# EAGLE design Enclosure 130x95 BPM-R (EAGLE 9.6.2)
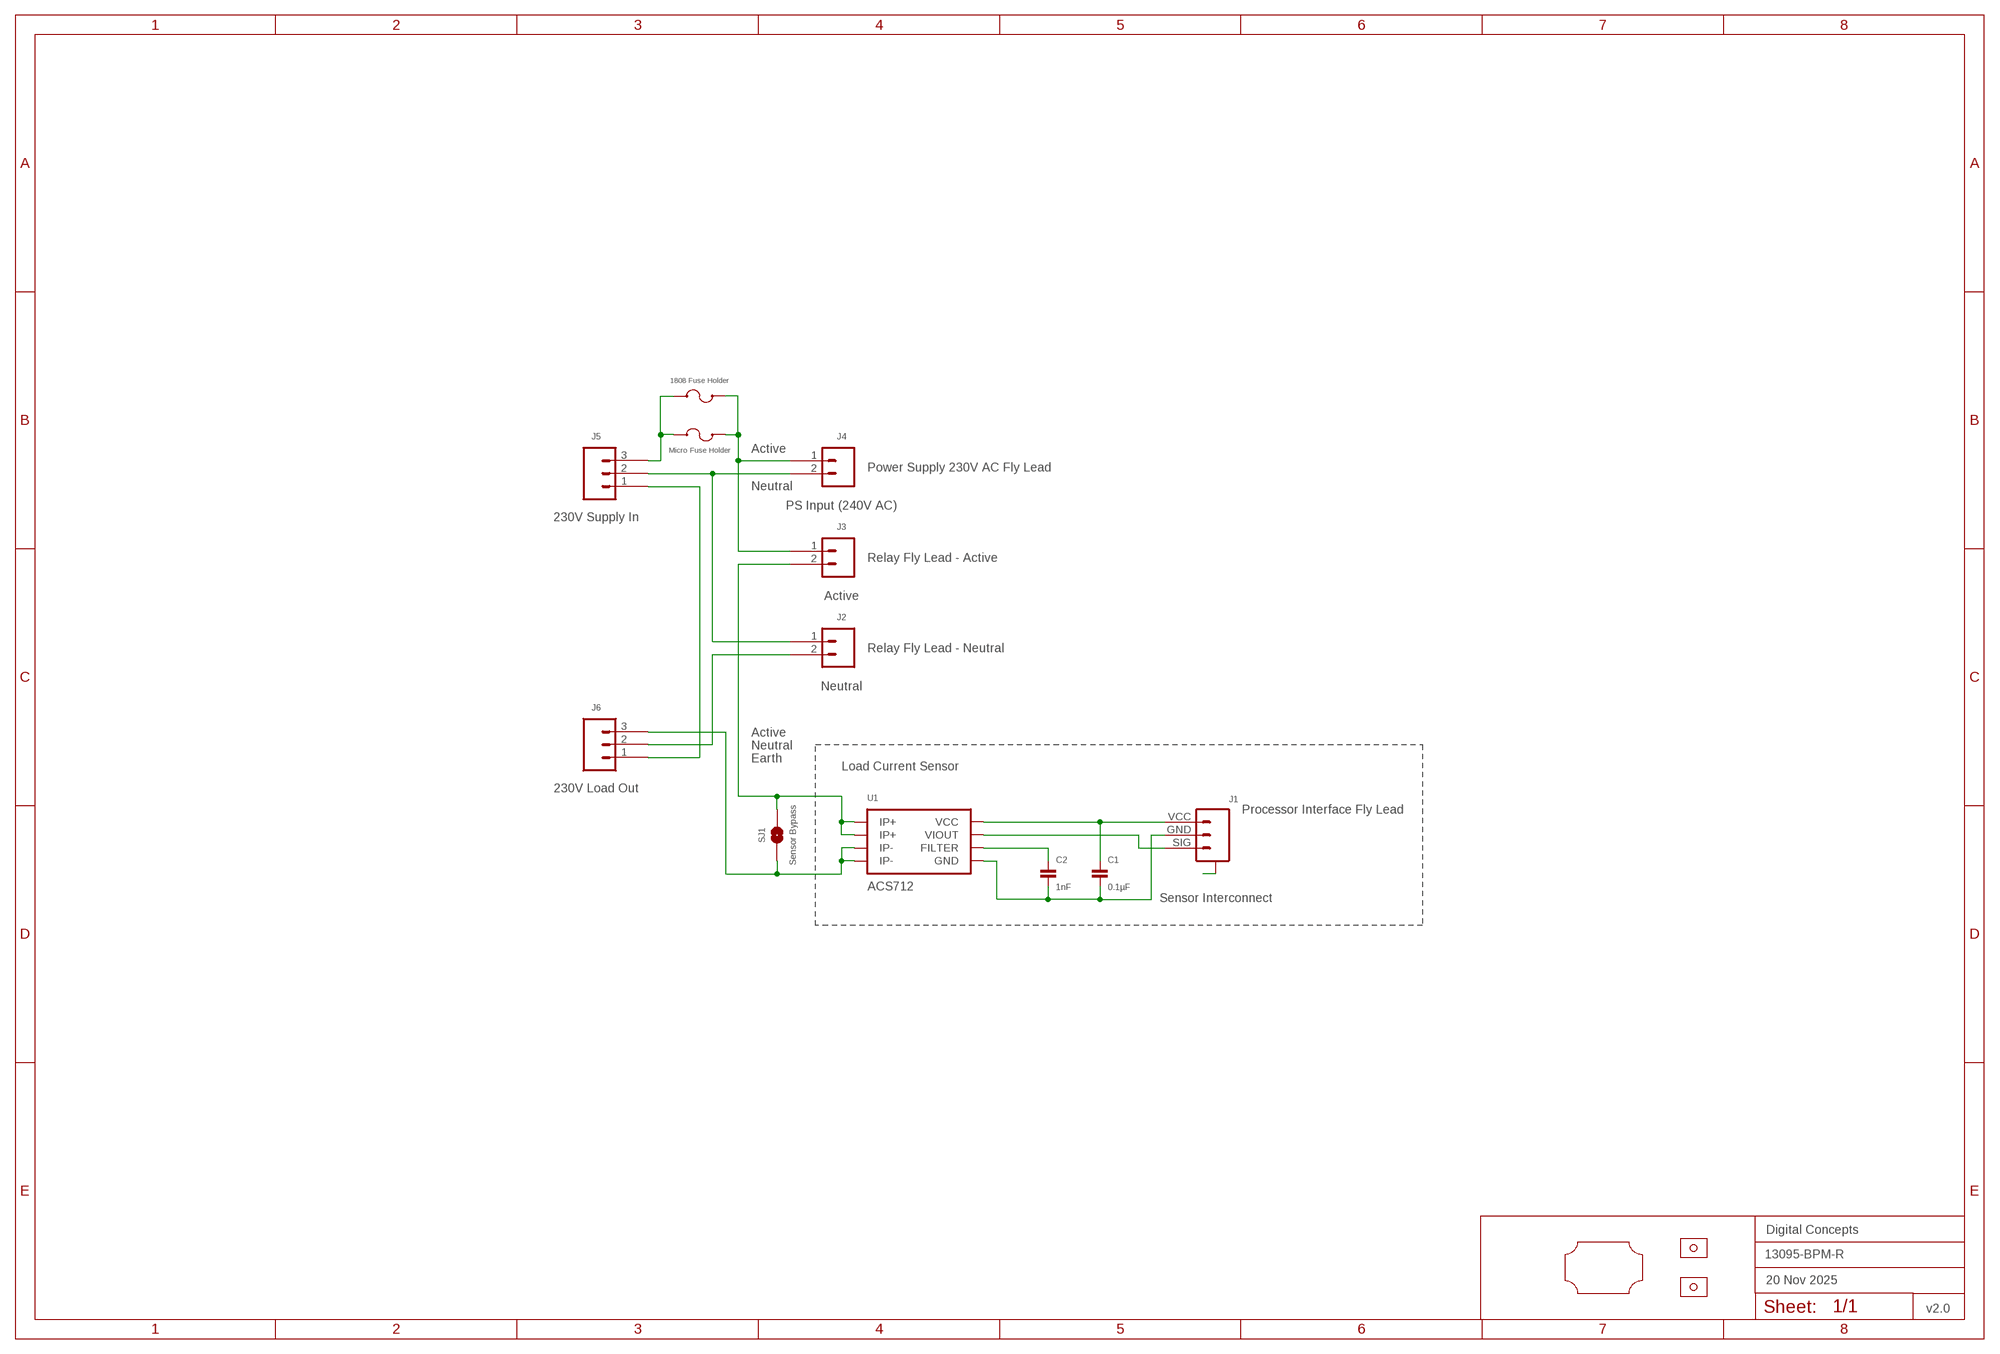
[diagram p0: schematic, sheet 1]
FRAME2 (A3L-LOC): DATE: 20 Nov 2025; OWNER: Digital Concepts; TITLE: 13095-BPM-R; VERSION: v2.0

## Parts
C1  0.1µF  CAPACITOR-0805  [C0805]
C2  1nF  CAPACITOR-0805  [C0805]
F2  1808 Fuse Holder  FUSE-HOLDER-1808  [FUSE-HOLDER-1808]
J1  Sensor Interconnect  JST-SH1.0-3-SMD-HORIZONTAL-SIG  [JST-SH1.0-3-HORIZONTAL-SIG]
J2  Neutral  TERMINAL_SCREW_2P_VERTICAL  [TERMINAL-SCREW-2P]
J3  Active  TERMINAL_SCREW_2P_VERTICAL  [TERMINAL-SCREW-2P]
J4  PS Input (240V AC)  JST-XH2.54-2-HORIZONTAL  [JST-XH2.4-2-HORIZONTAL]
J5  230V Supply In  TERMINAL_SCREW_3P_VERTICAL  [TERMINAL-SCREW-3P]
J6  230V Load Out  TERMINAL_SCREW_3P_VERTICAL  [TERMINAL-SCREW-3P]
SJ1  Sensor Bypass  SJ  [SJ]
U1  ACS712  [SOP-8]
U$1  PCB-OUTLINE-130X95-MAX-RC-H3  [PROTO-130X95-OUTLINE-MAX-RC-H3]
U$2  Micro Fuse Holder  FUSE-HOLDER  [FUSE-HOLDER-MICRO]
U$4  STRAIN-RELIEF-SADDLE  [STRAIN-RELIEF-SADDLE]
U$5  STRAIN-RELIEF-SADDLE  [STRAIN-RELIEF-SADDLE]

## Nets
A: J1.A@1(A) J1.A@3(A)
ACTIVE_IN: F2.P$2 J3.1 J4.1 U$2.P$3 U$2.P$4
ACTIVE_OUT: J3.2 SJ1.2 U1.1(IP+) U1.2(IP+)
EARTH: J5.1 J6.1
N$2: C1.1 J1.VCC U1.8(VCC)
N$3: J1.SIG U1.7(VIOUT)
N$7: F2.P$1 J5.3 U$2.P$1 U$2.P$2
N$19: J6.3 SJ1.1 U1.3(IP-) U1.4(IP-)
N$20: C1.2 C2.2 J1.GND U1.5(GND)
N$24: C2.1 U1.6(FILTER)
NEUTRAL_IN: J2.1 J4.2 J5.2
NEUTRAL_OUT: J2.2 J6.2

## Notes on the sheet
- Active
- Power Supply 230V AC Fly Lead
- Neutral
- Relay Fly Lead - Active
- Relay Fly Lead - Neutral
- Active
- Neutral
- Earth
- Load Current Sensor
- Processor Interface Fly Lead

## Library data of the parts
C1 C2 = digitalconcepts:CAPACITOR-0805: 0805 Capacitor
F2 = digitalconcepts:FUSE-HOLDER-1808: 1808 Fuse Holder
J1 = digitalconcepts:JST-SH1.0-3-SMD-HORIZONTAL-SIG: JST SH1.0 3P SMD Horizontal Connector with Signal
J2 J3 = digitalconcepts:TERMINAL_SCREW_2P_VERTICAL: PCB Mount Screw-Type Terminal 2P
J4 = digitalconcepts:JST-XH2.54-2-HORIZONTAL: XH2.54 2P Horizontal Connector
J5 J6 = digitalconcepts:TERMINAL_SCREW_3P_VERTICAL: PCB Mount Screw-Type Terminal 3P
SJ1 = digitalconcepts:SJ: Solder Jumper
U1 = digitalconcepts:ACS712: ACS712 Hall-Effect-Based Linear Current Sensor IC
U$1 = digitalconcepts:PCB-OUTLINE-130X95-MAX-RC-H3: PCB Eagle Max-Right-Cropped outline for 130 x 95 enclosure (Horizontal format)
U$2 = digitalconcepts:FUSE-HOLDER: Fuse Holder
U$4 U$5 = digitalconcepts:STRAIN-RELIEF-SADDLE: Strain Relief Saddle (7mm x 13mm)

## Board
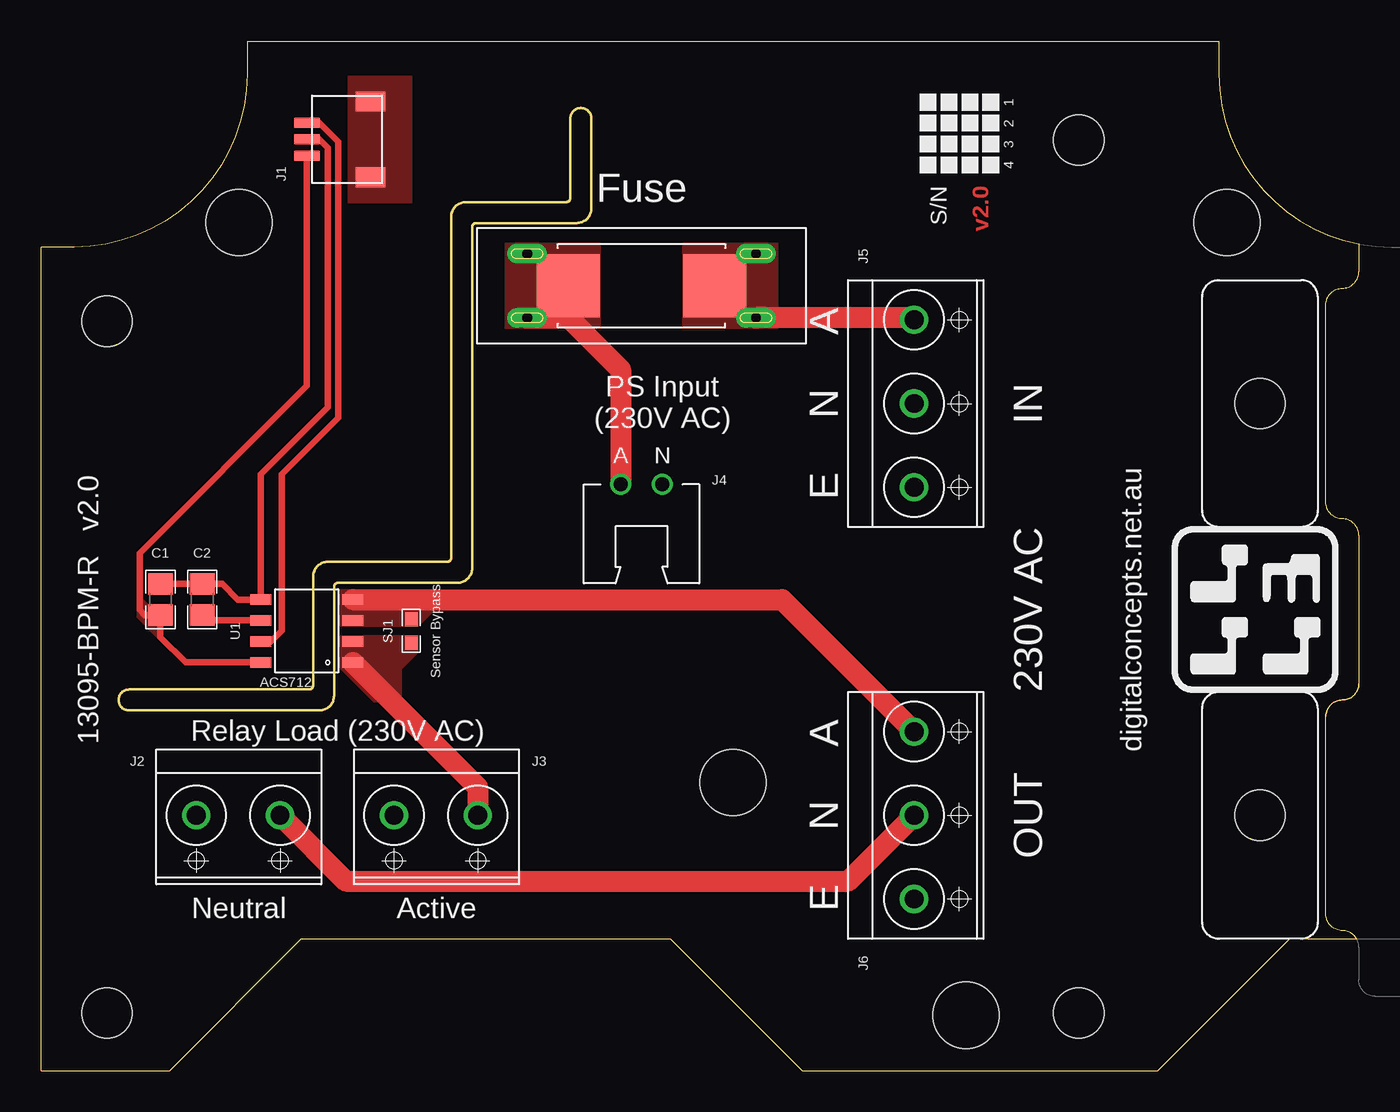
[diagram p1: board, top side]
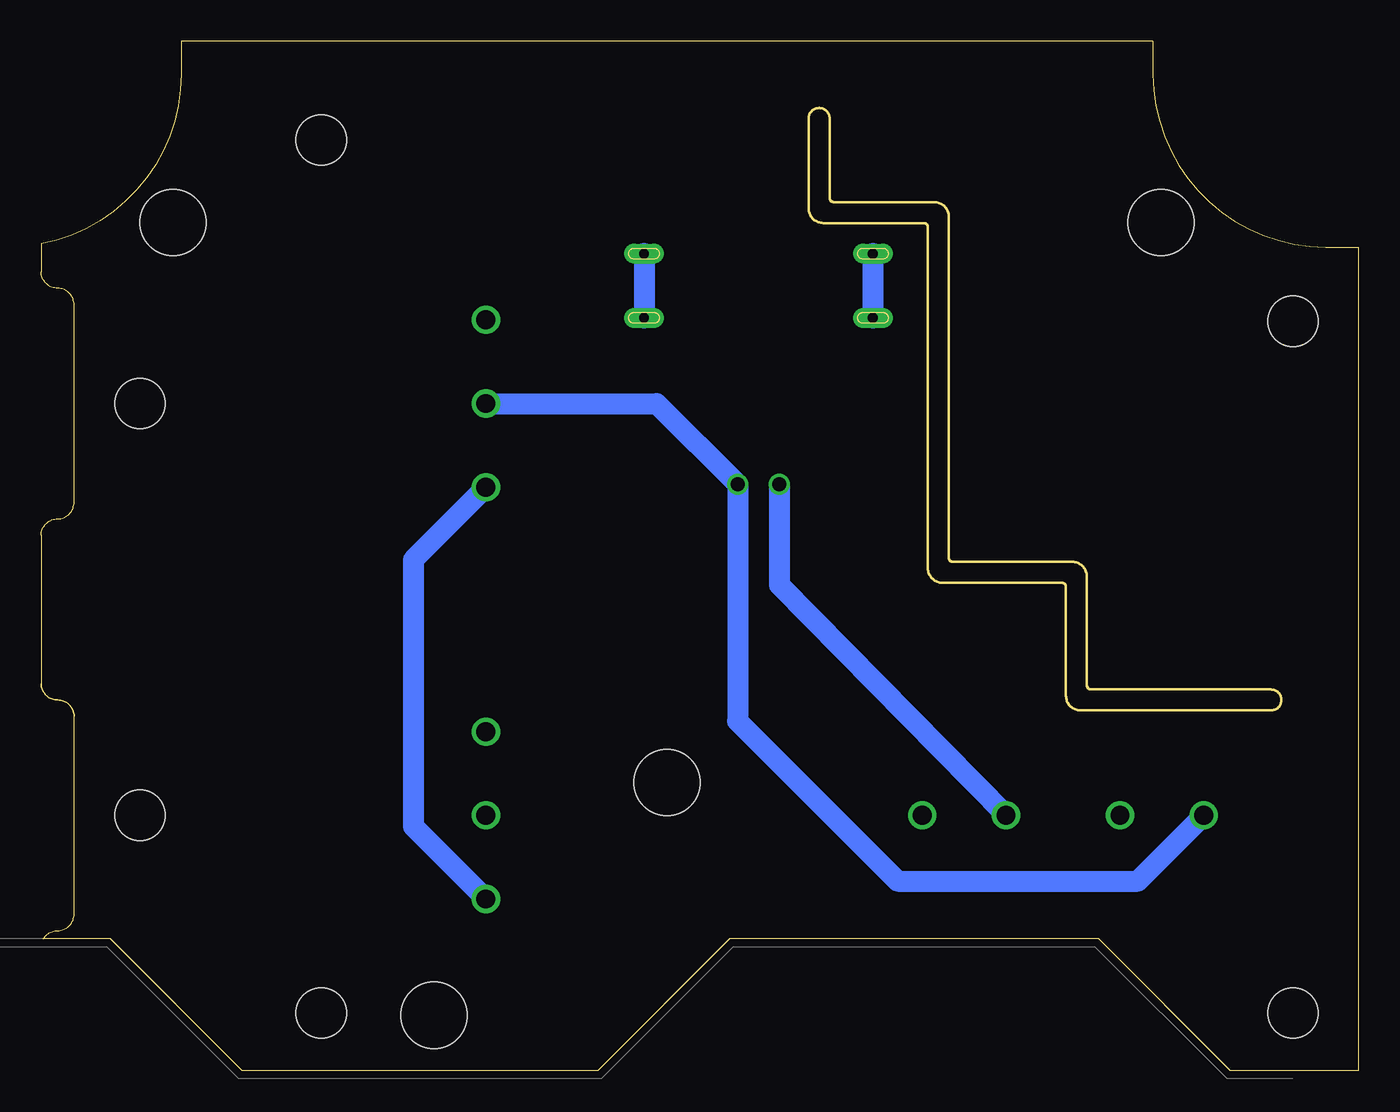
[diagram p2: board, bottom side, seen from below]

Size 80 x 62.5 mm. Coordinates in mm from the lower left corner, seen from the top.
Copper layers (1*16): Top 0.035mm / dielectric 1.5mm / Bottom 0.035mm
Design rules "default *": minimum track width 6mil, minimum drill 0.35mm, track to track 6mil, track to pad 6mil, pad to pad 6mil, via to via 6mil, smd to smd 6mil, copper to edge 6mil, drill to drill 6mil, minimum pad ring 1mil, minimum via ring 8mil, stop-mask expansion 4mil, vias tented up to drill 0mil, thermal gap 10mil
Milling: 24 lines

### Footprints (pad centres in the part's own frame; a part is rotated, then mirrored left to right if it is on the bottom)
C0805 = smd 1.3 x 1.5: 1 -0.95,0; 2 0.95,0
FUSE-HOLDER-1808 = smd 3.81 x 3.81: P$1 -4.445,0; P$2 4.445,0
JST-SH1.0-3-HORIZONTAL-SIG = smd 1.2 x 1.8: A@1 -2.3,-1.335; A@3 2.3,-1.335 | smd 0.6 x 1.55: GND 0,2.54; SIG 1,2.54; VCC -1,2.54
TERMINAL-SCREW-2P = drill 1.143: 1 -2.58,0; 2 2.5,0
JST-XH2.4-2-HORIZONTAL = drill 0.85: 1 1.27,0; 2 -1.27,0
TERMINAL-SCREW-3P = drill 1.143: 1 -5.08,0; 2 0,0; 3 5.08,0
SJ = smd 0.864 x 0.762: 1 -0.711,0; 2 0.711,0
SOP-8 = smd 0.635 x 1.27: 1 -1.905,-2.794; 2 -0.635,-2.794; 3 0.635,-2.794; 4 1.905,-2.794; 5 1.905,2.794; 6 0.635,2.794; 7 -0.635,2.794; 8 -1.905,2.794
PROTO-130X95-OUTLINE-MAX-RC-H3 = hole 3.048: -38,10; 21,21; 21,-32; -38,-32 | hole 4: 0,-18; -30,16; 30,16; 14.14,-32.14
FUSE-HOLDER-MICRO = drill 0.6 pad 1.2 long: P$1 -6.95,1.95; P$2 -6.95,-1.95; P$3 6.95,-1.95; P$4 6.95,1.95
STRAIN-RELIEF-SADDLE = hole 3.048: 0,0

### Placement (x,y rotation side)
C1  7.24,28.6 90 top
C2  9.78,28.6 90 top
F2  36.45,47.65 180 top
J1  18.67,56.54 90 top
J2  12,15.5 0 top
J3  24,15.5 0 top
J4  36.45,35.59 180 top
J5  53,40.5 90 top
J6  53,15.5 90 top
SJ1  22.48,26.7 270 top
U1  16.13,26.7 90 top
U$1  42,35.5 0 top
U$2  36.45,47.65 180 top
U$4  74,40.5 90 top
U$5  74,15.5 90 top

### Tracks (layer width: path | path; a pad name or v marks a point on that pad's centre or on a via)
A
  pour Top (no thermals): 18.67,60.35 22.48,60.35 22.48,52.73 18.67,52.73
ACTIVE_IN
  Top 1.27: U$2.P$4 32.04,45.7 35.18,42.56 J4.1
  Bottom 1.27: J4.1 35.18,29.49 J3.1 | U$2.P$3 U$2.P$4
  pour Top (no thermals): 28.2,50.19 33.91,50.19 33.91,45.11 28.2,45.11
ACTIVE_OUT
  Top 1.27: J3.2 26.5,17.21 U1.1
  pour Top (no thermals): 18.04,26.44 22.86,26.44 22.86,25.36 21.86,24.36 21.86,22.37 20.22,22.37 18.04,24.55
EARTH
  Bottom 1.27: J5.1 57.41,31.02 57.41,14.82 J6.1
N$2
  Top 0.406: U1.8 8.76,24.79 7.24,26.31 C1.1 6.29,27.65 5.97,27.97 5.97,31.41 16.13,41.57 J1.VCC
  pour Top (no thermals): 7.24,26.31 7.24,27.97 6.61,27.97 5.97,28.6 5.97,27.58
N$3
  Top 0.406: J1.SIG 16.89,57.54 18.04,56.4 18.04,39.65 14.61,36.22 14.61,26.7 13.97,26.06 U1.7
N$7
  Top 1.27: U$2.P$1 52.88,45.7 J5.3
  Bottom 1.27: U$2.P$2 U$2.P$1
  pour Top (no thermals): 38.99,50.19 44.7,50.19 44.7,45.11 38.99,45.11
N$19
  Top 1.27: J6.3 44.98,28.6 U1.4
  pour Top (no thermals): 18.04,29.23 23.75,29.23 24.38,28.6 24.38,28.47 22.86,26.95 18.04,26.95
N$20
  Top 0.406: C1.2 C2.2 10.99,29.55 11.94,28.6 U1.5 13.34,36.22 17.4,40.28 17.4,56.03 16.89,56.54 J1.GND
N$24
  Top 0.406: U1.6 10.1,27.33 C2.1
NEUTRAL_IN
  Bottom 1.27: J5.2 42.63,40.5 J4.2 37.72,21.22 28,11.5 13.42,11.5 J2.1
NEUTRAL_OUT
  Top 1.27: J2.2 18.5,11.5 49,11.5 J6.2

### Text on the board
Top: v2.0
tPlace: 1 | 2 | 3 | 4 | S/N | 13095-BPM-R v2.0 | digitalconcepts.net.au
tNames: Fuse | A | N | IN | PS Input / (230V AC) | A | N | E | 230V AC | Relay Load (230V AC) | A | N | OUT | E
